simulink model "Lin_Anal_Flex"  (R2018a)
settings: Solver=ode4  StartTime=0.0  StopTime=1  FixedStep=Ts  MaxStep=0.5  RelTol=1e-3  EnableMultiTasking=on
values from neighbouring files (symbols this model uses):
  Cw2b = [ 0,          0,          0    [run.m]
  Hco = [Hy0, 0, 0]'    [run.m]
  ini = [wb0; atto; Hco]    [run.m]
  Kq1 = I22*ww^2 - 3*wo2*(I11-I33)    [run.m]
  Kq2 = 2*I22*zet*ww    [run.m]
  Kqi = 0.0005    [run.m]
  Kr1 = (0.1*I11*I33*zet^2/Hy0) - sqrt( ((0.01^zet^4*I11^2*I33^2)/Hy0^2)+(4*I11*I33*zet^2) )    [run.m]
  Kr2 = 0.05*Kr1    [run.m]
  Kr3 = 0.04*zet*(Kr2-Hy0) * sqrt(abs(Hy0/(I11*I33)))    [run.m]
  nt = 7    [run.m]    (also in runf.m)
  Ts = 0.001    [run.m]    (also in runf.m = 0.0005)
  wo = Worb    [run.m]
undefined symbols (not defined in the file or in its folder): Avf, Bvf, Cvf, den, DiscIntNeverNeededParam, Dvf, num, RW_Steering, Spacecraft_Dynamics, Wheel_Dynamics
libraries: simulink x3

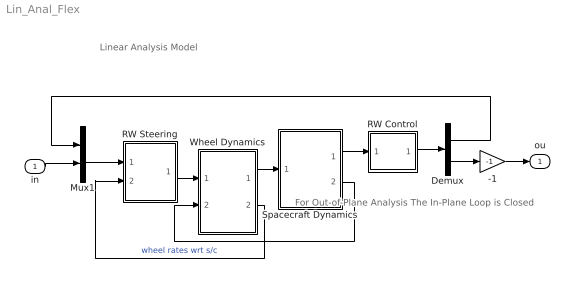
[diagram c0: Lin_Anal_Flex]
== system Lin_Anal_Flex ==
  note: Linear Analysis Model
  note: For Out-of-Plane Analysis The In-Plane Loop is Closed
  in : Inport
  -1 : Gain  Gain=-1
  Demux : Demux  Outputs=2
  Mux1 : Mux  Inputs=2
  RW Control : Subsystem
  RW Steering : Subsystem
  Spacecraft Dynamics : Subsystem
  Wheel Dynamics : Subsystem
  ou : Outport
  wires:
  Spacecraft Dynamics/1(atti) -> RW Control/1(atti)
  RW Control/1(Tc) -> Demux/1
  RW Steering/1(Twi) -> Wheel Dynamics/1(Twi)
  Wheel Dynamics/2(wr) -> RW Steering/2(wr(1))  "wheel rates wrt s/c"
  Mux1/1 -> RW Steering/1(Trwc)
  -1/1 -> ou/1
  Wheel Dynamics/1(Tcb) -> Spacecraft Dynamics/1(Trwa)
  Spacecraft Dynamics/2(wb) -> Wheel Dynamics/2(wb)
  in/1 -> Mux1/2
  Demux/2 -> -1/1
  Demux/1 -> Mux1/1

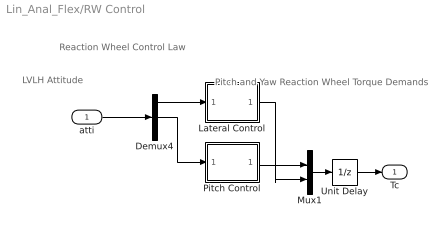
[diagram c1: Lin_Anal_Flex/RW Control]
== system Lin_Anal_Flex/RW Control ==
  note: Reaction Wheel Control Law
  note: LVLH Attitude
  note: Pitch and Yaw Reaction Wheel Torque Demands
  atti : Inport
  Demux4 : Demux  Outputs=3
  Lateral Control : Subsystem
  Mux1 : Mux  Inputs=2
  Pitch Control : Subsystem
  Unit Delay : UnitDelay  SampleTime=-1
  Tc : Outport
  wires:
  Mux1/1 -> Unit Delay/1
  Lateral Control/1(Tcz) -> Mux1/2
  atti/1 -> Demux4/1
  Demux4/2 -> Pitch Control/1(the)
  Pitch Control/1(Tcy) -> Mux1/1
  Demux4/1 -> Lateral Control/1(phi)
  Unit Delay/1 -> Tc/1

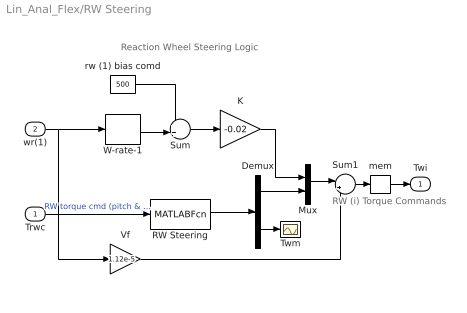
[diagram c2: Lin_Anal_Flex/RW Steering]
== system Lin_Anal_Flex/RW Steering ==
  note: Reaction Wheel Steering Logic
  note: RW (i) Torque Commands
  Trwc : Inport
  wr(1) : Inport  Port=2
  Demux : Demux  Outputs=[2, 1]
  K : Gain  Gain=-0.02
  Mux : Mux  Inputs=[1,2]
  RW Steering : MATLABFcn  MATLABFcn=RW_Steering( u(1:2) )  OutputDimensions=3
  Sum : Sum  Inputs=++|
  Sum1 : Sum  Inputs=|+-
  Twm : Scope
  Vf : Gain  Gain=1.12e-5
  W-rate-1 : Selector  InputPortWidth=3  IndexOptions=Index vector (dialog)  Indices=[1]  OutputSizes=1
  mem : Memory
  rw (1) bias comd : Constant  Value=500
  Twi : Outport
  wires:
  mem/1 -> Twi/1
  K/1 -> Mux/1
  W-rate-1/1 -> Sum/2
  rw (1) bias comd/1 -> Sum/1
  Sum/1 -> K/1
  wr(1)/1 -> Vf/1, W-rate-1/1
  Trwc/1 -> RW Steering/1  "RW torque cmd (pitch & yaw)"
  RW Steering/1 -> Demux/1
  Demux/1 -> Mux/2
  Demux/2 -> Twm/1
  Mux/1 -> Sum1/1
  Sum1/1 -> mem/1
  Vf/1 -> Sum1/2

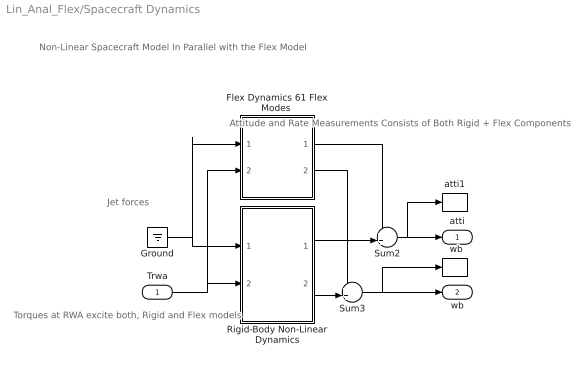
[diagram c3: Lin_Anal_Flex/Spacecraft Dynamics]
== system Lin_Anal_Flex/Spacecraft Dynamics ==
  note: Attitude and Rate Measurements Consists of Both Rigid + Flex Components
  note: Jet forces
  note: Torques at RWA excite both, Rigid and Flex models
  note: Non-Linear Spacecraft Model In Parallel with the Flex Model
  Trwa : Inport
  "  wb " : ToWorkspace  VariableName=wb  SampleTime=-1
  "Flex Dynamics 61 Flex Modes " : Subsystem
  Ground : Ground
  Rigid-Body Non-Linear Dynamics : Subsystem
  Sum2 : Sum  Inputs=++|
  Sum3 : Sum  Inputs=++|
  atti1 : ToWorkspace  VariableName=atti  SampleTime=-1
  atti : Outport
  wb : Outport  Port=2
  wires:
  Sum3/1 -> "  wb "/1, wb/1
  Sum2/1 -> atti1/1, atti/1
  "Flex Dynamics 61 Flex Modes "/2(wb-flx) -> Sum3/1
  Rigid-Body Non-Linear Dynamics/2(wbr) -> Sum3/2
  Rigid-Body Non-Linear Dynamics/1(atti) -> Sum2/2
  "Flex Dynamics 61 Flex Modes "/1(att-flx) -> Sum2/1
  Trwa/1 -> Rigid-Body Non-Linear Dynamics/2(Tcb), "Flex Dynamics 61 Flex Modes "/2(Trwi)
  Ground/1 -> Rigid-Body Non-Linear Dynamics/1(Frcs), "Flex Dynamics 61 Flex Modes "/1(Frcs)

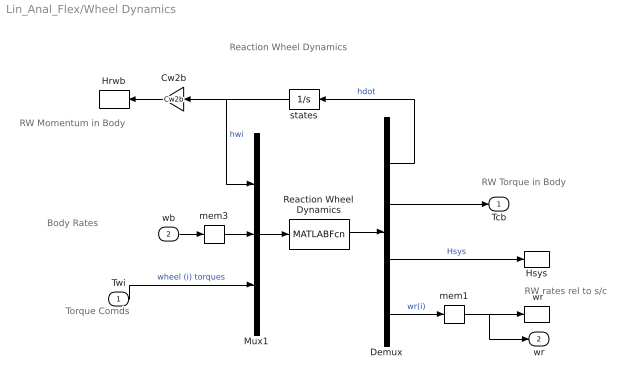
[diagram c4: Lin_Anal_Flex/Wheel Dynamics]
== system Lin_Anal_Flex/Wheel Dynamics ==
  note: RW Momentum in Body
  note: Torque Comds
  note: RW rates rel to s/c
  note: RW Torque in Body
  note: Body Rates
  note: Reaction Wheel Dynamics
  Twi : Inport
  wb : Inport  Port=2
  " wr" : ToWorkspace  VariableName=wr  SampleTime=-1
  Cw2b : Gain  Gain=Cw2b  Multiplication=Matrix(K*u)
  Demux : Demux  Outputs=[3, 3, 3, 3]
  Hrwb : ToWorkspace  VariableName=Hrwb  SampleTime=-1
  Hsys : ToWorkspace  VariableName=Hsys  SampleTime=-1
  Mux1 : Mux  Inputs=[3, 3, 3]
  Reaction Wheel Dynamics : MATLABFcn  MATLABFcn=Wheel_Dynamics( u(1:3), u(4:6), u(7:9) )  OutputDimensions=3+3+3+3
  mem1 : Memory  InheritSampleTime=on
  mem3 : Memory  InheritSampleTime=on
  states : Integrator  InitialCondition=Hco
  Tcb : Outport
  wr : Outport  Port=2
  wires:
  mem1/1 -> wr/1, " wr"/1
  mem3/1 -> Mux1/2
  Twi/1 -> Mux1/3  "wheel (i) torques"
  Demux/2 -> Tcb/1
  Reaction Wheel Dynamics/1 -> Demux/1
  Mux1/1 -> Reaction Wheel Dynamics/1
  wb/1 -> mem3/1
  Demux/4 -> mem1/1  "wr(i)"
  Demux/3 -> Hsys/1  "Hsys"
  Demux/1 -> states/1  "hdot"
  Cw2b/1 -> Hrwb/1
  states/1 -> Mux1/1, Cw2b/1  "hwi"

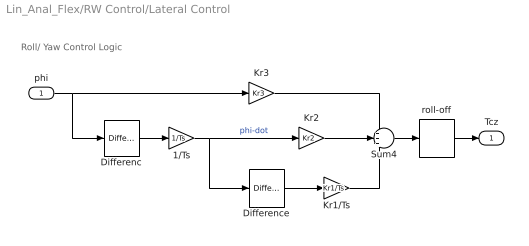
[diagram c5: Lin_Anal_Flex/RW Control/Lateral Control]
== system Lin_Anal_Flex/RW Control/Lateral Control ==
  note: Roll/ Yaw Control Logic
  phi : Inport
  1/Ts : Gain  Gain=1/Ts
  Differenc : simulink/Discrete/Difference  ICPrevInput=0.0  InputProcessing=Inherited  OutMin=[]  OutMax=[]  OutDataType=sfix(16)  OutScaling=2^-10  DoSatur=off
  Difference : simulink/Discrete/Difference  ICPrevInput=0.0  InputProcessing=Inherited  OutMin=[]  OutMax=[]  OutDataType=sfix(16)  OutScaling=2^-10  DoSatur=off
  Kr1/Ts : Gain  Gain=Kr1/Ts
  Kr2 : Gain  Gain=Kr2
  Kr3 : Gain  Gain=Kr3
  Sum4 : Sum  Inputs=+++
  roll-off : DiscreteTransferFcn  Numerator=[num]  Denominator=[den]  SampleTime=Ts
  Tcz : Outport
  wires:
  1/Ts/1 -> Difference/1, Kr2/1  "phi-dot"
  Differenc/1 -> 1/Ts/1
  Difference/1 -> Kr1/Ts/1
  Sum4/1 -> roll-off/1
  phi/1 -> Differenc/1, Kr3/1
  Kr1/Ts/1 -> Sum4/3
  Kr2/1 -> Sum4/2
  Kr3/1 -> Sum4/1
  roll-off/1 -> Tcz/1

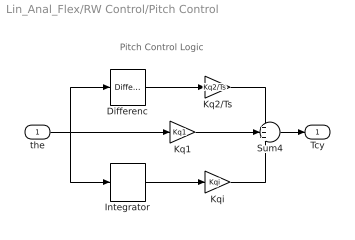
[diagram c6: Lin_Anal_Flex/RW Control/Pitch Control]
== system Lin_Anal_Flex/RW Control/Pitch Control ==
  note: Pitch Control Logic
  the : Inport
  Differenc : simulink/Discrete/Difference  ICPrevInput=0.0  InputProcessing=Inherited  OutMin=[]  OutMax=[]  OutDataType=sfix(16)  OutScaling=2^-10  DoSatur=off
  Integrator : DiscreteIntegrator  SampleTime=Ts  ICPrevOutput=DiscIntNeverNeededParam  ICPrevScaledInput=DiscIntNeverNeededParam
  Kq1 : Gain  Gain=Kq1
  Kq2/Ts : Gain  Gain=Kq2/Ts
  Kqi : Gain  Gain=Kqi
  Sum4 : Sum  Inputs=+++
  Tcy : Outport
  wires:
  Differenc/1 -> Kq2/Ts/1
  Integrator/1 -> Kqi/1
  Kqi/1 -> Sum4/3
  the/1 -> Differenc/1, Integrator/1, Kq1/1
  Kq2/Ts/1 -> Sum4/1
  Sum4/1 -> Tcy/1
  Kq1/1 -> Sum4/2

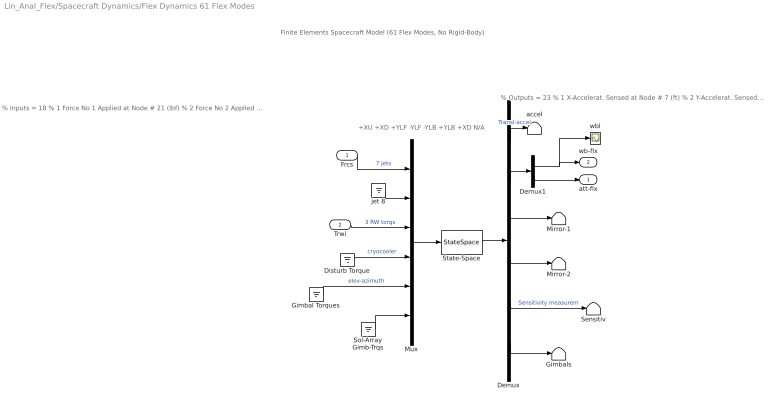
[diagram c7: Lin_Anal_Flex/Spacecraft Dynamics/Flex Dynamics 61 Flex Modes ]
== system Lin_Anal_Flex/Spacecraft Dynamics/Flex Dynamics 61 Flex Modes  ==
  note: Finite Elements Spacecraft Model (61 Flex Modes, No Rigid-Body)
  note: % Inputs = 18 % 1 Force No 1 Applied at Node # 21 (lbf) % 2 Force No 2 Applied at Node # 22 (lbf) % 3 Force No 3 Applied at Node # 23 (lbf) % 4 Force No 4 Applied at Node # 24 (lbf) % 5 Force No 5 Applied at Node # 25 (lbf) % 6 Force No 6 Applied at Node # 26 (lbf) % 7 Force No 7 Applied at Node # 27 (lbf) % 8 Force No 8 Applied at Node # 28 (lbf) % 9 Torque No 1 Applied at Node # 17 (ft-lb) % 10 Torque No 2 Applied at Node # 18 (ft-lb) % 11 Torque No 3 Applied at Node # 19 (ft-lb) % 12 Torque No 4 Applied at Node # 8 (ft-lb) % 13 Torque No 5 Applied at Node # 8 (ft-lb) % 14 Torque No 6 Applied at Node # 8 (ft-lb) % 15 Control Torque at Gimbal No 1 in (ft-lb) % 16 Control Torque at Gimbal No 2 in (ft-lb) % 17 Control Torque at Gimbal No 3 in (ft-lb) % 18 Control Torque at Gimbal No 4 in (ft-lb)
  note: % Outputs = 23 % 1 X-Accelerat. Sensed at Node # 7 (ft) % 2 Y-Accelerat. Sensed at Node # 7 (ft) % 3 X-Rot. Rate Sensed at Node # 6 (radian) % 4 Y-Rot. Rate Sensed at Node # 6 (radian) % 5 Z-Rot. Rate Sensed at Node # 6 (radian) % 6 X-Rotation Sensed at Node # 6 (radian) % 7 Y-Rotation Sensed at Node # 6 (radian) % 8 Z-Rotation Sensed at Node # 6 (radian) % 9 Y-Rotation Sensed at Node # 9 (radian) % 10 Z-Rotation Sensed at Node # 9 (radian) % 11 Y-Rotation Sensed at Node # 10 (radian) % 12 Z-Rotation Sensed at Node # 10 (radian) % 13 X-Rotation Sensed at Node # 11 (radian) % 14 Y-Rotation Sensed at Node # 12 (radian) % 15 Z-Rotation Sensed at Node # 13 (radian) % 16 Rotation Angle at Gimbal No 1 in (radians) % 17 Rotation Rate at Gimbal No 1 in (rad/sec) % 18 Rotation Angle at Gimbal No 2 in (radians) % 19 Rotation Rate at Gimbal No 2 in (rad/sec) % 20 Rotation Angle at Gimbal No 3 in (radians) % 21 Rotation Rate at Gimbal No 3 in (rad/sec) % 22 Rotation Angle at Gimbal No 4 in (radians) % 23 Rotation Rate at Gimbal No 4 in (rad/sec)
  note: +XU +XD +YLF -YLF -YLB +YLB +XD N/A
  Frcs : Inport
  Trwi : Inport  Port=2
  Demux : Demux  Outputs="[2, 6, 2,2,3,  8]"
  Demux1 : Demux  Outputs=[3, 3]
  Disturb Torque : Ground
  Gimbal Torques : Ground
  Gimbals : Terminator
  Mirror-1 : Terminator
  Mirror-2 : Terminator
  Mux : Mux  Inputs=[7,1,3,3,2,2]
  Sensitiv : Terminator
  Sol-Array Gimb-Trqs : Ground
  State-Space : StateSpace  A=Avf  B=Bvf  C=Cvf  D=Dvf  InitialCondition=0
  accel : Terminator
  jet 8 : Ground
  wbl : Scope
  att-flx : Outport
  wb-flx : Outport  Port=2
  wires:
  Demux/6 -> Gimbals/1
  Gimbal Torques/1 -> Mux/5  "elev-azimuth"
  Demux/1 -> accel/1  "Transl-accel"
  State-Space/1 -> Demux/1
  Demux/2 -> Demux1/1
  Demux1/1 -> wbl/1, wb-flx/1
  Mux/1 -> State-Space/1
  Frcs/1 -> Mux/1  "7 Jets"
  jet 8/1 -> Mux/2
  Trwi/1 -> Mux/3  "3 RW torqs"
  Disturb Torque/1 -> Mux/4  "cryocooler"
  Sol-Array Gimb-Trqs/1 -> Mux/6
  Demux/5 -> Sensitiv/1  "Sensitivity measurem"
  Demux/3 -> Mirror-1/1
  Demux/4 -> Mirror-2/1
  Demux1/2 -> att-flx/1

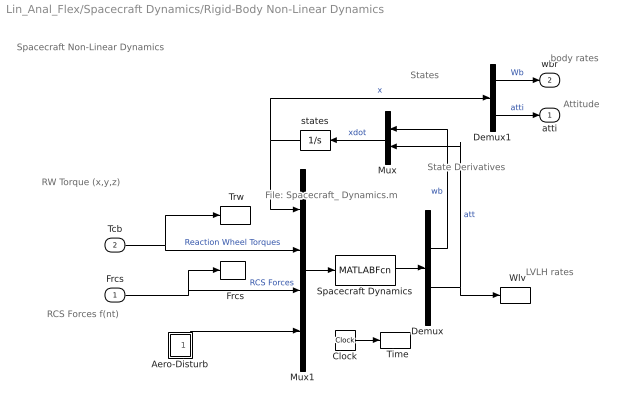
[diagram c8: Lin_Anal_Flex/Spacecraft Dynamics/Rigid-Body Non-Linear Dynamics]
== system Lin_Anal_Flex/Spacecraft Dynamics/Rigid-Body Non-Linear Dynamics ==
  note: File: Spacecraft_ Dynamics.m
  note: Attitude
  note: LVLH rates
  note: RW Torque (x,y,z)
  note: States
  note: RCS Forces f(nt)
  note: body rates
  note: State Derivatives
  note: Spacecraft Non-Linear Dynamics
  Frcs : Inport  PortDimensions=nt
  Tcb : Inport  Port=2
  "  Frcs" : ToWorkspace  VariableName=Frcs  SampleTime=-1
  "  Time" : ToWorkspace  VariableName=time  SampleTime=-1
  "  Wlv" : ToWorkspace  VariableName=wlv  SampleTime=-1
  " Trw" : ToWorkspace  VariableName=Trwb  SampleTime=-1
  Aero-Disturb : Subsystem
  Clock : Clock
  Demux : Demux  Outputs=[3,3]
  Demux1 : Demux  Outputs=[3,3]
  Mux : Mux  Inputs=[3,3]
  Mux1 : Mux  Inputs=[6, 3, nt, 3]
  Spacecraft Dynamics : MATLABFcn  MATLABFcn=Spacecraft_Dynamics( u(1:6), u(7:9), u(10:9+nt), u(10+nt:12+nt) )  OutputDimensions=6
  states : Integrator  InitialCondition=ini
  atti : Outport
  wbr : Outport  Port=2
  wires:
  Aero-Disturb/1(Td) -> Mux1/4
  Tcb/1 -> " Trw"/1, Mux1/2  "Reaction Wheel Torques"
  Demux1/2 -> atti/1  "atti"
  Demux1/1 -> wbr/1  "Wb"
  Spacecraft Dynamics/1 -> Demux/1
  Mux1/1 -> Spacecraft Dynamics/1
  Demux/1 -> Mux/1  "wb"
  Demux/2 -> "  Wlv"/1, Mux/2  "att"
  states/1 -> Mux1/1, Demux1/1  "x"
  Frcs/1 -> Mux1/3, "  Frcs"/1  "RCS Forces"
  Clock/1 -> "  Time"/1
  Mux/1 -> states/1  "xdot"

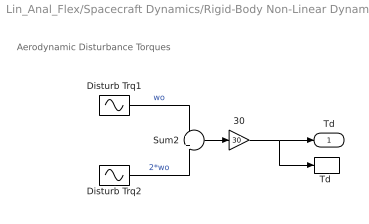
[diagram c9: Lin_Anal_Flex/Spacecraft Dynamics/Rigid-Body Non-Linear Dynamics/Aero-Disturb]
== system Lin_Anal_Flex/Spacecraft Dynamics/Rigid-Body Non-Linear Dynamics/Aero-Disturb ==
  note: Aerodynamic Disturbance Torques
  30 : Gain  Gain=30
  Disturb Trq1 : Sin  Amplitude="[0.0,   1,   0.2]*0.0001"  Bias="[0.0,  0.5,  0.15]*0.0001"  Frequency=[wo, wo, wo]  SampleTime=0
  Disturb Trq2 : Sin  Amplitude=[0, 1.2, 1]*0.0001  Bias=[0 0 0]  Frequency=[wo, wo, wo]*2  SampleTime=0
  Sum2 : Sum  Inputs=+|+
  "Td " : ToWorkspace  VariableName=Td  SampleTime=-1
  Td : Outport
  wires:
  Disturb Trq1/1 -> Sum2/1  "wo"
  Sum2/1 -> 30/1
  Disturb Trq2/1 -> Sum2/2  "2*wo"
  30/1 -> Td/1, "Td "/1
